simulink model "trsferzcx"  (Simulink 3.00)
settings: Solver=ode45  SolverMode=SingleTasking  StartTime=0.0  StopTime=10.0  RelTol=1e-3  AbsTol=1e-6

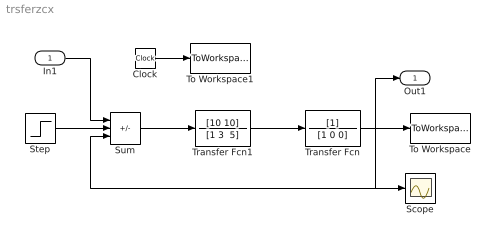
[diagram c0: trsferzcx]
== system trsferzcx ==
  In1 : Inport  Port=1  PortWidth=-1  SampleTime=-1  DataType=auto
  Clock : Clock
  Scope : Scope
  Step : Step  Time=1  Before=0  After=1  SampleTime=0
  Sum : Sum  Inputs=++-  SaturateOnIntegerOverflow=on
  To Workspace : ToWorkspace  VariableName=y  SampleTime=-1  SaveFormat=Matrix
  To Workspace1 : ToWorkspace  VariableName=t  SampleTime=-1  SaveFormat=Matrix
  Transfer Fcn : TransferFcn  Numerator=[1]  Denominator=[1 0 0]
  Transfer Fcn1 : TransferFcn  Numerator=[10 10]  Denominator="[1 3  5]"
  Out1 : Outport  Port=1
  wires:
  Sum/1 -> Transfer Fcn1/1
  Transfer Fcn1/1 -> Transfer Fcn/1
  Transfer Fcn/1 -> To Workspace/1, Sum/3, Scope/1, Out1/1
  Step/1 -> Sum/2
  In1/1 -> Sum/1
  Clock/1 -> To Workspace1/1
